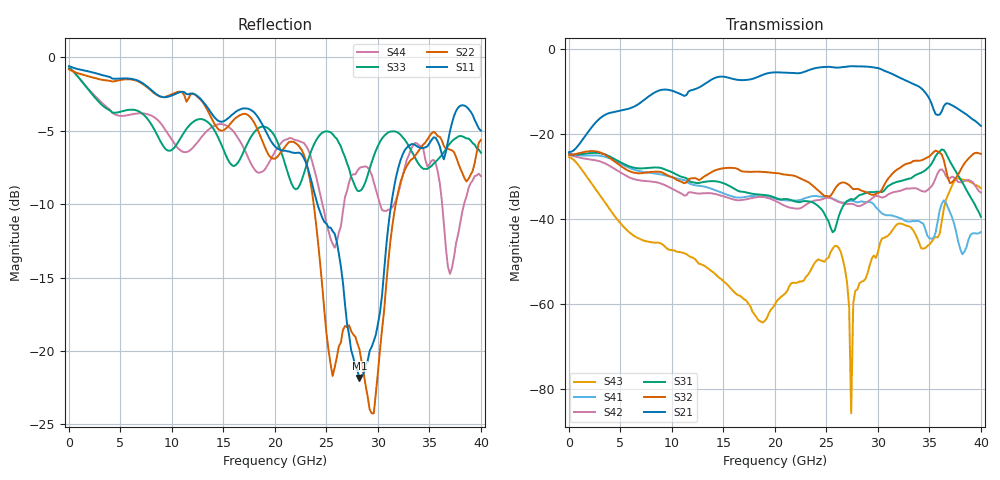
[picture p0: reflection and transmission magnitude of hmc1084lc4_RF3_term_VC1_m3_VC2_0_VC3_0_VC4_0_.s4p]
!Agilent Technologies,N5224A,MY51441122,A.09.40.06
!Agilent N5224A: A.09.40.06
!Date: Thursday, June 19, 2014 00:49:55
!Correction: S11(Full 4 Port(1,2,3,4))
!S12(Full 4 Port(1,2,3,4))
!S13(Full 4 Port(1,2,3,4))
!S14(Full 4 Port(1,2,3,4))
!S21(Full 4 Port(1,2,3,4))
!S22(Full 4 Port(1,2,3,4))
!S23(Full 4 Port(1,2,3,4))
!S24(Full 4 Port(1,2,3,4))
!S31(Full 4 Port(1,2,3,4))
!S32(Full 4 Port(1,2,3,4))
!S33(Full 4 Port(1,2,3,4))
!S34(Full 4 Port(1,2,3,4))
!S41(Full 4 Port(1,2,3,4))
!S42(Full 4 Port(1,2,3,4))
!S43(Full 4 Port(1,2,3,4))
!S44(Full 4 Port(1,2,3,4))
!S4P File: Measurements: <S11,S12,S13,S14>,
!<S21,S22,S23,S24>,
!<S31,S32,S33,S34>,
!<S41,S42,S43,S44>:
# Hz S  dB  R 50
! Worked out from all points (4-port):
!   201 points, 10 MHz to 40 GHz, reference 50 ohm
!   strongest paths, dB at 10 MHz, 10.01 GHz, 20 GHz, 30 GHz, 40 GHz:
!     S21: -24.2, -9.8, -5.4, -4.4, -18.1
!     S32: -24.8, -30.1, -29.2, -33.9, -24.7
!     S31: -24.7, -29.0, -35.0, -33.6, -39.5
!     S42: -24.9, -32.9, -35.7, -34.6, -33.8
!     S41: -24.9, -30.2, -35.2, -37.7, -43.1
!     S43: -25.4, -47.3, -60.1, -47.8, -32.8
!   lowest |S11| = -21.8 dB at 28.2 GHz (marker M1), VSWR 1.18, Z = 55.8 - j6.32 ohm
!   |S11| at or under -10 dB: 24.13 GHz to 31.3 GHz (7.17 GHz wide, 25.9 % of centre)
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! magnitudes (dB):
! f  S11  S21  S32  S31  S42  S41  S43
! 10 MHz  -0.6  -24.2  -24.8  -24.7  -24.9  -24.9  -25.4
! 18.81 GHz  -4.6  -6.0  -28.9  -34.3  -34.8  -34.8  -64.4
! 26 GHz  -12.6  -4.3  -32.3  -41.0  -35.8  -35.7  -46.4
! 27 GHz  -18.2  -4.1  -31.7  -35.8  -36.5  -35.9  -55.0
! 27.4 GHz  -20.0  -4.0  -32.5  -35.3  -36.4  -35.7  -85.8
! 28.2 GHz  -21.8  -4.0  -33.1  -34.4  -37.0  -36.0  -55.2
! 40 GHz  -5.0  -18.1  -24.7  -39.5  -33.8  -43.1  -32.8
